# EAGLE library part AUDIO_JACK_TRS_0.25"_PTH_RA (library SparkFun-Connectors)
Audio Jack, 1/4" TRS jack, horizontal, PTH, aka "Phono jack" Find the connector here: Audio Jack - 1/4" Stereo (right angle) (COM-11144) Datasheet Note, although the datasheet and physical part are slightly different, this footprint was proven to mate well on the Proto Pedal. This device is used on these SparkFun Products: SparkFun TRS Jack Breakout - 1/4" Stereo (BOB-13005 ) SparkFun Proto Pedal - sorry bad link - product comming soon! (PRT-13124)
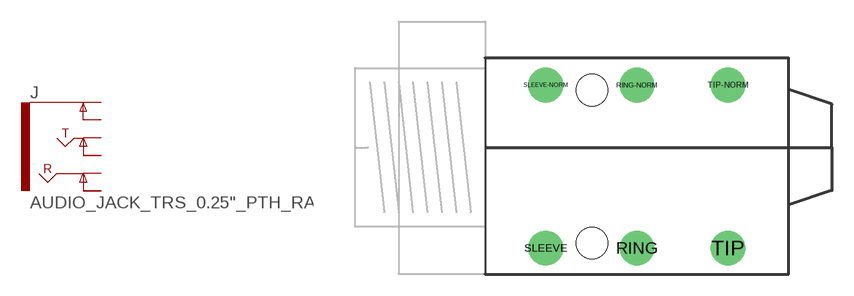
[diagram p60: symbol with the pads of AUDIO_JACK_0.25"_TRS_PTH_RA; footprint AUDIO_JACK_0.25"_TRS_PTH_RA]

Designator prefix J

## AUDIO_JACK_TRS_0.25"_PTH_RA (PROD_ID: CONN-12339; SF_ID: COM-11144)  [AUDIO_JACK_0.25"_TRS_PTH_RA]
RING  RING
RING-NORM  RING-NORM
SLEEVE  EARTH
SLEEVE-NORM  EARTH-NORM
TIP  TIP
TIP-NORM  TIP-NORM

## Footprint AUDIO_JACK_0.25"_TRS_PTH_RA (pad centres in mm)
Right Angle -1/4" Stereo Jack Specifications: Pin count: 6 Datasheet referenced for footprint Example device(s): AUDIO_JACK_TRS_0.25"_PTH_RA
drill 1.6: RING 10.5,-6.95; RING-NORM 10.5,4.35; SLEEVE 4.2,-6.95; SLEEVE-NORM 4.2,4.35; TIP 16.8,-6.95; TIP-NORM 16.8,4.35
hole 2.2 at 7.4,4
hole 2.2 at 7.4,-6.6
